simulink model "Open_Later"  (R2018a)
settings: Solver=ode45  StartTime=0.0  StopTime=10  RelTol=1e-3  EnableMultiTasking=on
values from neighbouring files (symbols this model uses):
  Aact = [0, 1; -omg^2, -2*zet*omg]    [init.m]
  Bact = [0; omg^2]    [init.m]
  Cact = [1,0]    [init.m]
  Cyb = -0.0245    [init.m]    (also in lqr_des.m)
  Cydel = [-0.24668,0.24668, 0.47413,-0.47413,0]/100    [init.m]    (also in lqr_des.m = [-0.24668,0.24668, 0.47413,-0.47413]/100)
  d2r = pi/180    (= 0.0174532925199)    [init.m]
  Dact = 0    [init.m]
  Mass = 198.32    [init.m]    (also in lqr_des.m)
  Qbar = 150    [init.m]    (also in lqr_des.m)
  r2d = 180/pi    (= 57.2957795131)    [init.m]    (also in pl.m)
  Sref = 79.069    [init.m]    (also in lqr_des.m)
undefined symbols (not defined in the file or in its folder): Ap, Bp, Cp, Dp, Kmix, Kpr

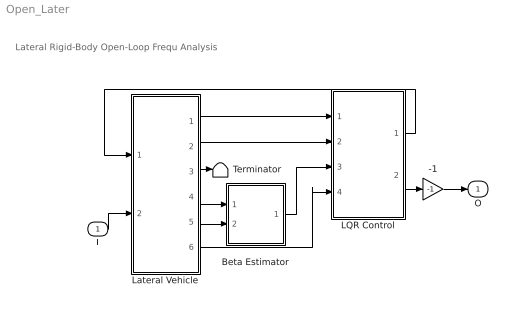
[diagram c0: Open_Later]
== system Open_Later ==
  note: Lateral Rigid-Body Open-Loop Frequ Analysis
  I : Inport
  -1 : Gain  Gain=-1
  Beta Estimator : Subsystem
  LQR Control : Subsystem
  Lateral Vehicle : Subsystem
  Terminator : Terminator
  O : Outport
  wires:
  Lateral Vehicle/1(p) -> LQR Control/1(p)
  Lateral Vehicle/2(r) -> LQR Control/2(r)
  Lateral Vehicle/6(phi) -> LQR Control/4(phi)
  -1/1 -> O/1
  Lateral Vehicle/4(delta) -> Beta Estimator/1(delta)
  Lateral Vehicle/5(Ny) -> Beta Estimator/2(Ydd)
  Lateral Vehicle/3(beta) -> Terminator/1
  Beta Estimator/1(bethat) -> LQR Control/3(beta)
  I/1 -> Lateral Vehicle/2(dR)
  LQR Control/2(dR) -> -1/1
  LQR Control/1(dP) -> Lateral Vehicle/1(dP)

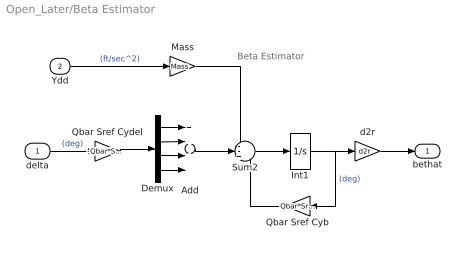
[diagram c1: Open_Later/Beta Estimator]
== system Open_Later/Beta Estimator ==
  note: Beta Estimator
  delta : Inport
  Ydd : Inport  Port=2
  Add : Sum  Inputs=++++
  Demux : Demux
  Int1 : Integrator
  Mass : Gain  Gain=Mass
  Qbar Sref Cyb : Gain  Gain=Qbar*Sref*Cyb
  Qbar Sref Cydel : Gain  Gain=-Qbar*Sref*Cydel
  Sum2 : Sum  Inputs=--+
  d2r : Gain  Gain=d2r
  bethat : Outport
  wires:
  Add/1 -> Sum2/2
  d2r/1 -> bethat/1
  Mass/1 -> Sum2/1
  Ydd/1 -> Mass/1  "(ft/sec^2)"
  Qbar Sref Cyb/1 -> Sum2/3
  Int1/1 -> d2r/1, Qbar Sref Cyb/1  "(deg)"
  Sum2/1 -> Int1/1
  delta/1 -> Qbar Sref Cydel/1  "(deg)"
  Qbar Sref Cydel/1 -> Demux/1
  Demux/1 -> Add/1
  Demux/2 -> Add/2
  Demux/3 -> Add/3
  Demux/4 -> Add/4

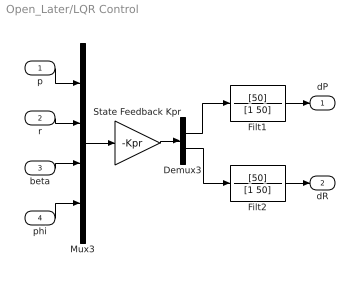
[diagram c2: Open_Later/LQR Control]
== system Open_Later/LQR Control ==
  p : Inport
  r : Inport  Port=2
  beta : Inport  Port=3
  phi : Inport  Port=4
  Demux3 : Demux  Outputs=2
  Filt1 : TransferFcn  Numerator=[50]  Denominator=[1 50]
  Filt2 : TransferFcn  Numerator=[50]  Denominator=[1 50]
  Mux3 : Mux
  State Feedback Kpr : Gain  Gain=-Kpr  Multiplication=Matrix(K*u) (u vector)
  dP : Outport
  dR : Outport  Port=2
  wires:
  Filt2/1 -> dR/1
  Filt1/1 -> dP/1
  Demux3/2 -> Filt2/1
  phi/1 -> Mux3/4
  beta/1 -> Mux3/3
  Demux3/1 -> Filt1/1
  r/1 -> Mux3/2
  p/1 -> Mux3/1
  Mux3/1 -> State Feedback Kpr/1
  State Feedback Kpr/1 -> Demux3/1

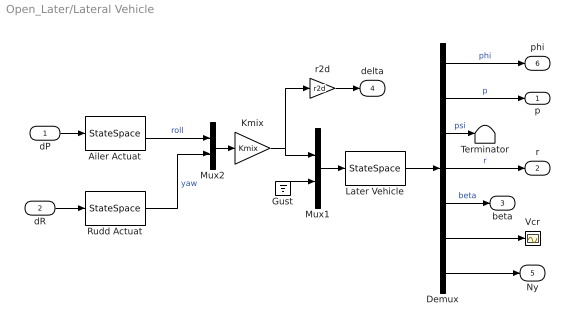
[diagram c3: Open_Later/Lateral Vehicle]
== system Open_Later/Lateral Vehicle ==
  dP : Inport
  dR : Inport  Port=2
  Ailer Actuat : StateSpace  A=Aact  B=Bact  C=Cact  D=Dact  InitialCondition=0
  Demux : Demux  Outputs=7
  Gust : Ground
  Kmix : Gain  Gain=Kmix  Multiplication=Matrix(K*u) (u vector)
  Later Vehicle : StateSpace  A=Ap  B=Bp  C=Cp  D=Dp  InitialCondition=0
  Mux1 : Mux  Inputs=[4,1]
  Mux2 : Mux  Inputs=2
  Rudd Actuat : StateSpace  A=Aact  B=Bact  C=Cact  D=Dact  InitialCondition=0
  Terminator : Terminator
  Vcr : Scope
  r2d : Gain  Gain=r2d
  p : Outport
  r : Outport  Port=2
  beta : Outport  Port=3
  delta : Outport  Port=4
  Ny : Outport  Port=5
  phi : Outport  Port=6
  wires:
  Demux/7 -> Ny/1
  Demux/6 -> Vcr/1
  dR/1 -> Rudd Actuat/1
  Demux/4 -> r/1  "r"
  dP/1 -> Ailer Actuat/1
  Demux/2 -> p/1  "p"
  Demux/1 -> phi/1  "phi"
  Demux/5 -> beta/1  "beta"
  Later Vehicle/1 -> Demux/1
  Mux2/1 -> Kmix/1
  Rudd Actuat/1 -> Mux2/2  "yaw"
  Kmix/1 -> Mux1/1, r2d/1
  Mux1/1 -> Later Vehicle/1
  Ailer Actuat/1 -> Mux2/1  "roll"
  Gust/1 -> Mux1/2
  r2d/1 -> delta/1
  Demux/3 -> Terminator/1  "psi"
